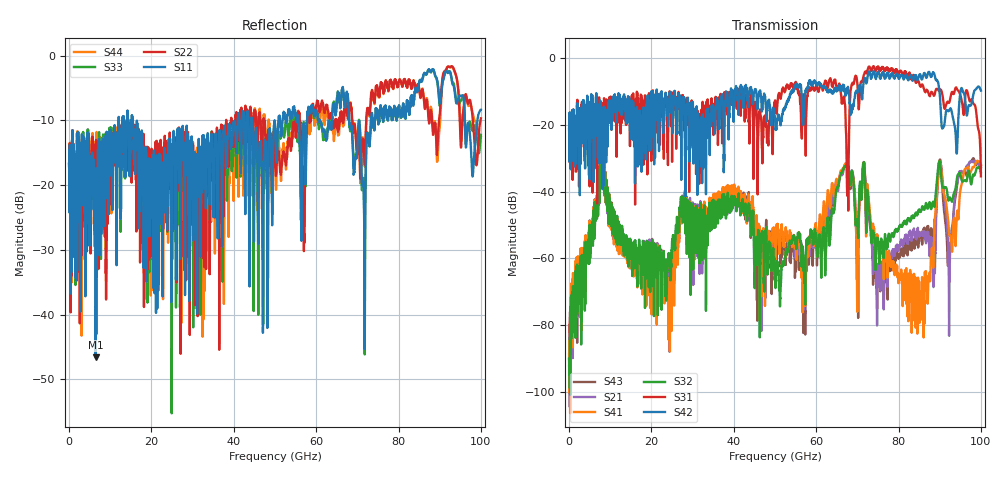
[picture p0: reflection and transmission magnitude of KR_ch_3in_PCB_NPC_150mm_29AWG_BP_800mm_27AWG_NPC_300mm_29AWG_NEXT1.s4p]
# GHz S RI R 45
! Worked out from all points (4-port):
!   4000 points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, 25 MHz to 100 GHz, reference 45 ohm
!   strongest paths, dB at 25 MHz, 25.02 GHz, 50.02 GHz, 75.03 GHz, 100 GHz:
!     S42: -21.3, -17.5, -18.0, -4.3, -9.8
!     S31: -21.2, -31.1, -12.8, -2.5, -35.5
!     S32: -90.1, -54.8, -65.1, -55.4, -34.3
!     S41: -88.7, -64.7, -62.6, -54.3, -31.9
!     S21: -90.2, -60.0, -58.1, -64.1, -32.8
!     S43: -92.2, -59.1, -54.7, -63.9, -32.3
!   lowest |S11| = -46.6 dB at 6.475 GHz (marker M1), VSWR 1.01, Z = 45.1 - j0.418 ohm
!   |S11| at or under -10 dB: start of sweep to 12.07 GHz; 15.43 GHz to 40.98 GHz (25.55 GHz wide, 90.6 % of centre); 44.43 GHz to 49.9 GHz (5.471 GHz wide, 11.6 % of centre)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
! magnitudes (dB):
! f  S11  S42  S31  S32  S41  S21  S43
! 25 MHz  -16.7  -21.3  -21.2  -90.1  -88.7  -90.2  -92.2
! 6.475 GHz  -46.6  -17.0  -24.1  -45.6  -45.3  -45.8  -45.1
! 57.12 GHz  -11.9  -14.0  -10.9  -67.5  -68.0  -70.5  -67.9
! 67.3 GHz  -6.4  -10.5  -23.0  -32.0  -31.5  -31.7  -31.7
! 85.8 GHz  -3.6  -6.2  -8.1  -44.4  -68.3  -53.1  -54.9
! 90 GHz  -7.3  -10.7  -9.8  -30.9  -31.4  -31.7  -30.5
! 100 GHz  -8.3  -9.8  -35.5  -34.3  -31.9  -32.8  -32.3
